TYPE STR_APC :
STRUCT
	Outputs_Valve_Default_Control_Mode_7100_13						:	USINT	;
	Outputs_Process_Controller_Process_Setpoint_7050_13				:	REAL	;
	Outputs_Valve_Default_Position_Setpoint_7100_12					:	REAL	;
	Outputs_Process_Controller_Exh_Rate_5050_01						:	REAL	;
	Outputs_Process_Controller_Active_Controller_7050_11			:	USINT	;
	Outputs_Process_Controller_Slow_exhaust_control_arriva_4050_01	:	REAL	;
	Inputs_Sensor_Input_Defau_Value_6030_11							:	REAL	;
	Inputs_Sensor_Input_Defau_Value_6040_11							:	REAL	;
	Inputs_Valve_Default_Position_Actual_Value_6100_11				:	REAL	;
	Inputs_Valve_Default_Control_Mode_Status_6100_14				:	USINT	;
	Inputs_Valve_Default_Homing_Status_6100_15						:	USINT	;
	Inputs_Process_Controller_Selected_Controller_6050_14			:	USINT	;
	Inputs_Active_Device_Warni_SubIndex_001_F381_01					:	UDINT	;
	Inputs_Active_Device_Warni_SubIndex_003_F381_03					:	UDINT	;
	Inputs_Active_Device_Warni_SubIndex_004_F381_04					:	UDINT	;
	Inputs_Active_Device_Warni_SubIndex_005_F381_05					:	UDINT	;
	Inputs_Active_Device_Warni_SubIndex_016_F381_10					:	UDINT	;
	Inputs_Active_Manufacturer_SubIndex_016_F382_10					:	UDINT	;
	Inputs_Active_Manufacturer_SubIndex_001_F384_01					:	UDINT	;
	Inputs_Active_Manufacturer_SubIndex_003_F384_03					:	UDINT	;
	Inputs_Active_Manufacturer_SubIndex_004_F384_04					:	UDINT	;
	Inputs_Active_Manufacturer_SubIndex_016_F384_10					:	UDINT	;	
END_STRUCT
END_TYPE
